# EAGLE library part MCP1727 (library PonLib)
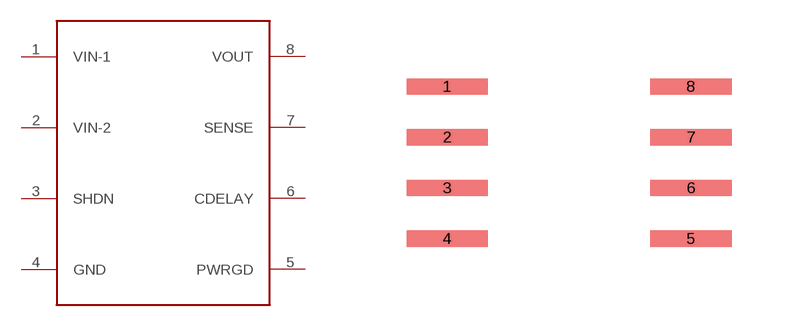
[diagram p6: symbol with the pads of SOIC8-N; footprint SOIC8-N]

Designator prefix -

## MCP1727  [SOIC8-N]
1  VIN-1
2  VIN-2
3  SHDN
4  GND
5  PWRGD
6  CDELAY
7  SENSE
8  VOUT

## Footprint SOIC8-N (pad centres in mm)
smd 2.032 x 0.406: 1 -3.048,1.905; 2 -3.048,0.635; 3 -3.048,-0.635; 4 -3.048,-1.905; 5 3.048,-1.905; 6 3.048,-0.635; 7 3.048,0.635; 8 3.048,1.905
